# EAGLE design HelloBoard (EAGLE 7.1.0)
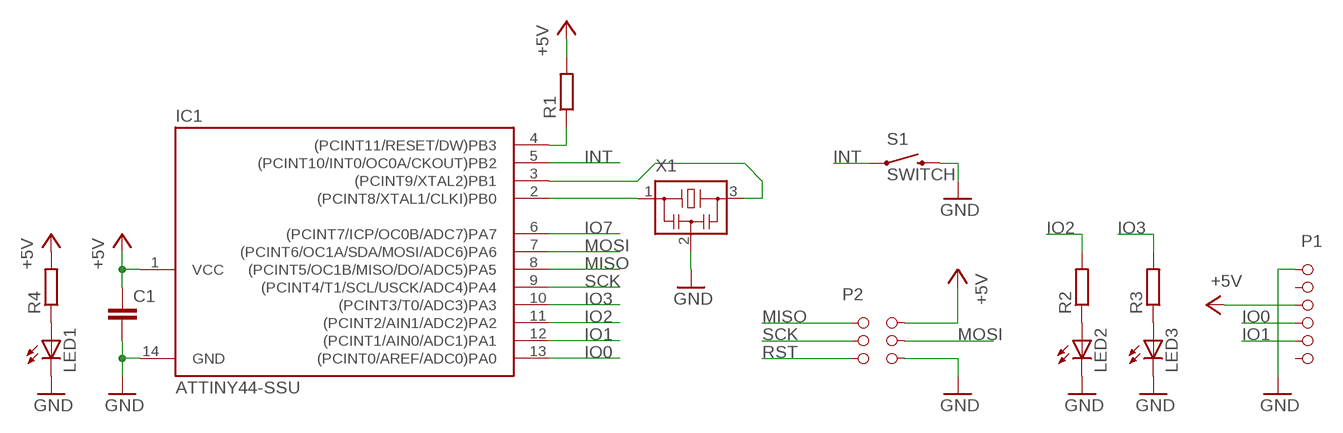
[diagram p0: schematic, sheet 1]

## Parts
C1  C-EUC1206  [C1206]
IC1  ATTINY44-SSU  [SOIC14]
LED1  LEDSMT1206  [1206]
LED2  LEDSMT1206  [1206]
LED3  LEDSMT1206  [1206]
P1  SMD-6  [SMD-6]
P2  SMD-3-2  [SMD-3-2]
R1  R-EU_R1206  [R1206]
R2  R-EU_R1206  [R1206]
R3  R-EU_R1206  [R1206]
R4  R-EU_R1206  [R1206]
S1  SWITCH  SWITCH-MOMENTARY-2-SMD-1101NE  [TACTILE-SWITCH-1101NE]
X1  RESONATOR-PBRC  [PBRC]

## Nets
+5V: C1.1 IC1.1(VCC) P1.P$3 P2.1 R1.2 R4.2
GND: C1.2 IC1.14(GND) LED1.C LED2.C LED3.C P1.P$1 P2.3 S1.2 X1.2
INT: IC1.5((PCINT10/INT0/OC0A/CKOUT)PB2) S1.1
IO0: IC1.13((PCINT0/AREF/ADC0)PA0) P1.P$4
IO1: IC1.12((PCINT1/AIN0/ADC1)PA1) P1.P$5
IO2: IC1.11((PCINT2/AIN1/ADC2)PA2) R2.2
IO3: IC1.10((PCINT3/T0/ADC3)PA3) R3.2
IO7: IC1.6((PCINT7/ICP/OC0B/ADC7)PA7)
MISO: IC1.8((PCINT5/OC1B/MISO/DO/ADC5)PA5) P2.6
MOSI: IC1.7((PCINT6/OC1A/SDA/MOSI/ADC6)PA6) P2.2
N$1: IC1.2((PCINT8/XTAL1/CLKI)PB0) X1.1
N$2: IC1.3((PCINT9/XTAL2)PB1) X1.3
N$3: LED2.A R2.1
N$4: LED3.A R3.1
N$5: LED1.A R4.1
RST: IC1.4((PCINT11/RESET/DW)PB3) P2.4 R1.1
SCK: IC1.9((PCINT4/T1/SCL/USCK/ADC4)PA4) P2.5
Unconnected: P1.P$2 P1.P$6

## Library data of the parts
C1 = rcl:C-EU: CAPACITOR, European symbol
IC1 = fab:ATTINY44
LED1-LED3 = led:LED: LED
P1 = PinHeader:SMD-6
P2 = PinHeader:SMD-3-2
R1-R4 = rcl:R-EU_: RESISTOR, European symbol
S1 = SparkFun-Electromechanical:SWITCH-MOMENTARY-2: Various NO switches- pushbuttons, reed, etc
X1 = fab:RESONATOR-PBRC

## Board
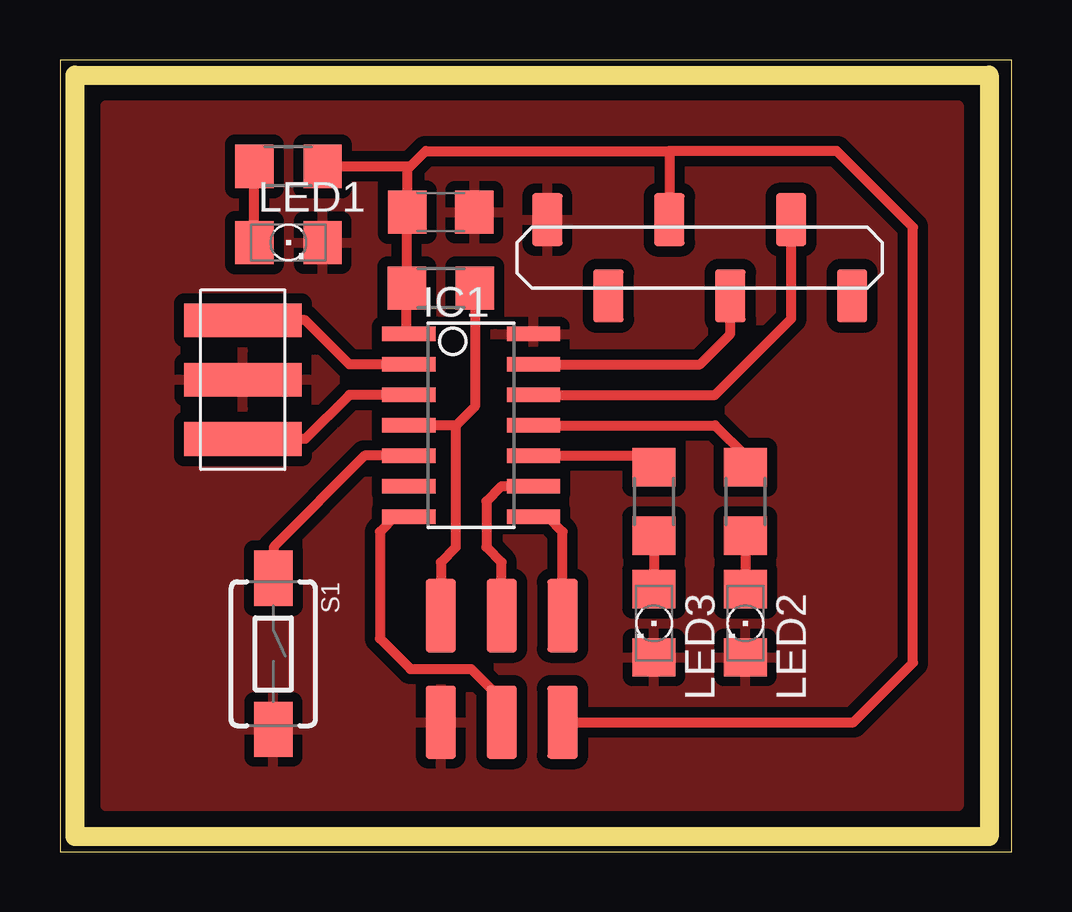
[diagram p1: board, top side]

Size 39.67 x 33.01 mm. Coordinates in mm from the lower left corner, seen from the top.
Outline: 0,0 39.67,0 39.67,33.01 0,33.01 0,0
Copper layers (1*16): Top 0.035mm / dielectric 1.5mm / Bottom 0.035mm
Design rules "default *": minimum track width 10mil, minimum drill 24mil, track to track 16mil, track to pad 16mil, pad to pad 16mil, via to via 8mil, smd to smd 8mil, copper to edge 40mil, drill to drill 8mil, minimum pad ring 10mil, minimum via ring 8mil, stop-mask expansion 0mil, vias tented up to drill 0mil, thermal gap 16mil
Milling: 4 lines

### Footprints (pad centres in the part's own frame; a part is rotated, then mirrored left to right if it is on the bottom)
C1206 = smd 1.6 x 1.8: 1 -1.4,0; 2 1.4,0
SOIC14 = smd 0.61 x 2.21: 1 -3.81,-2.603; 2 -2.54,-2.603; 3 -1.27,-2.603; 4 0,-2.603; 5 1.27,-2.603; 6 2.54,-2.603; 7 3.81,-2.603; 8 3.81,2.603; 9 2.54,2.603; 10 1.27,2.603; 11 0,2.603; 12 -1.27,2.603; 13 -2.54,2.603; 14 -3.81,2.603
1206 = smd 1.6 x 1.803: A -1.422,0; C 1.422,0
SMD-6 = smd 1.27 x 2.2: P$1 -6.35,1.587; P$2 -3.81,-1.587; P$3 -1.27,1.587; P$4 1.27,-1.587; P$5 3.81,1.587; P$6 6.35,-1.587
SMD-3-2 = smd 1.27 x 3.048: 1 -2.54,2.223; 2 0,2.223; 3 2.54,2.223; 4 2.54,-2.223; 5 0,-2.223; 6 -2.54,-2.223
R1206 = smd 1.6 x 1.803: 1 -1.422,0; 2 1.422,0
TACTILE-SWITCH-1101NE = smd 2.3 x 1.6: 1 -3.15,0; 2 3.15,0
PBRC = smd 1.4 x 4.9: 1 -2.475,0; 2 0,0; 3 2.475,0

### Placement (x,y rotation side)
C1  15.88,26.67 0 top
IC1  17.14,17.78 270 top
LED1  9.53,25.4 0 top
LED2  28.57,9.53 270 top
LED3  24.77,9.53 270 top
P1  26.67,24.77 0 top
P2  18.41,7.62 180 top
R1  15.88,23.5 180 top
R2  28.57,14.61 90 top
R3  24.77,14.61 90 top
R4  9.53,28.57 0 top
S1  8.89,8.26 270 top
X1  7.62,19.68 270 top

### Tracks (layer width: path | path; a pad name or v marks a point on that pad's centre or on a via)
+5V
  Top 0.406: IC1.1 14.45,21.59 R1.2 14.45,26.04 C1.1 14.47,28.45 14.61,28.57 | P2.1 33.08,5.4 35.56,7.88 35.56,26.04 32.38,29.21 25.4,29.21 | 25.4,29.21 15.24,29.21 14.61,28.57 | 25.4,29.21 P1.P$3 | R4.2 14.61,28.57
GND
  pour Top (isolate 0.432): 1.91,31.11 37.47,31.11 37.47,1.91 1.91,1.91
INT
  Top 0.406: IC1.5 12.7,16.51 8.91,12.7 S1.1
IO0
  Top 0.406: IC1.13 26.67,20.32 27.94,21.59 P1.P$4
IO1
  Top 0.406: IC1.12 27.3,19.05 30.48,22.23 P1.P$5
IO2
  Top 0.406: IC1.11 27.3,17.78 28.57,16.51 R2.2
IO3
  Top 0.406: IC1.10 24.28,16.51 R3.2
MISO
  Top 0.406: IC1.8 20.32,13.97 20.95,13.34 P2.6
MOSI
  Top 0.406: IC1.7 13.97,13.97 13.34,13.34 13.34,8.89 14.61,7.62 17.14,7.62 18.41,6.35 P2.2
N$1
  Top 0.406: IC1.2 12.06,20.32 10.22,22.16 X1.1
N$2
  Top 0.406: IC1.3 12.06,19.05 10.22,17.21 X1.3
N$3
  Top 0.406: R2.1 LED2.A
N$4
  Top 0.406: R3.1 LED3.A
N$5
  Top 0.406: LED1.A R4.1
RST
  Top 0.406: 16.51,17.78 16.51,12.7 15.88,12.06 P2.4 | 16.51,17.78 IC1.4 | R1.1 17.3,18.57 16.51,17.78
SCK
  Top 0.406: IC1.9 18.41,15.24 17.78,14.61 17.78,12.7 18.41,12.06 P2.5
